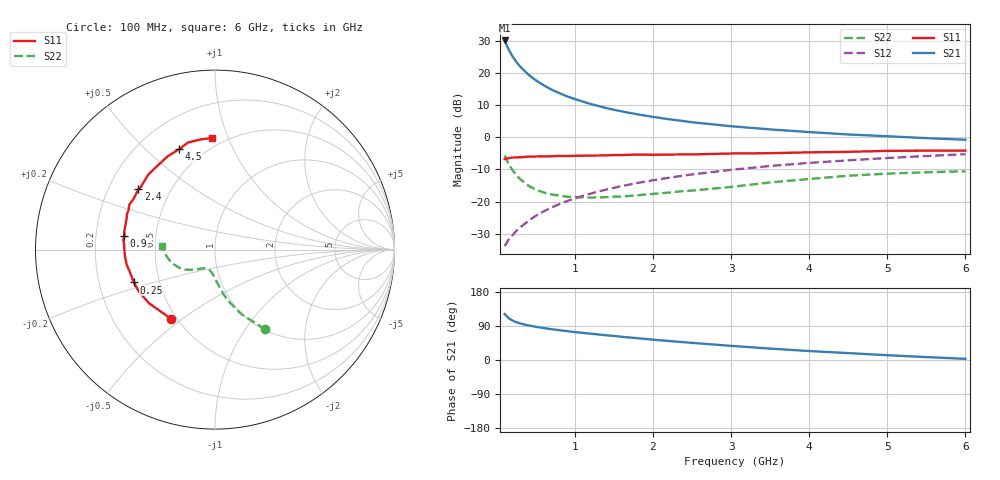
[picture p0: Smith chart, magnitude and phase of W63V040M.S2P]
! SIEMENS Small Signal Semiconductors
! BFR193W
! Si NPN RF Bipolar Junction Transistor in SOT323
! VCE = 3 V  IC = 40 mA
! Common Emitter S-Parameters:  September  1992
# GHz  S  MA  R  50
!  f  S11  S21  S12  S22
! GHz  MAG  ANG  MAG  ANG  MAG  ANG  MAG  ANG
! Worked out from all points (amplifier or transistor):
!   28 points, 100 MHz to 6 GHz, reference 50 ohm
!   highest |S21| = 30.2 dB at 100 MHz (marker M1)
!   |S21| within 3 dB of that: start of sweep to 156.1 MHz
!   unconditionally stable (mu >= 1): 556.4 MHz to 2.38 GHz; 2.431 GHz to 2.542 GHz
!   at 300 MHz: K = 0.90, MSG = 25.0 dB, |S12| = -28.0 dB
!   at 1.5 GHz: K = 1.03, MAG = 11.1 dB, |S12| = -15.7 dB
!   at 6 GHz: K = 0.92, MSG = 2.2 dB, |S12| = -5.3 dB
!   S11 on the Smith chart (normalised r, x): 100 MHz: 0.47, -0.46; 250 MHz: 0.36, -0.17; 900 MHz: 0.32, +0.07; 2.4 GHz: 0.33, +0.31; 4.5 GHz: 0.37, +0.64; 6 GHz: 0.43, +0.88
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0.1  0.4569 -122.2  32.18 121.4  0.0202 60.0  0.5249 -57.8
0.15  0.4739 -141.0  23.49 110.8  0.0254 60.5  0.3886 -67.8
0.2  0.4841 -151.0  18.31 104.2  0.0297 62.5  0.3096 -74.1
0.25  0.4877 -158.0  14.93 99.8  0.0349 64.3  0.2562 -79.0
0.3  0.4887 -163.2  12.61 96.4  0.0396 66.2  0.223 -81.9
0.4  0.4993 -170.6  9.556 91.4  0.0494 68.9  0.1781 -87.1
0.5  0.5026 -175.5  7.703 87.6  0.06 70.4  0.1527 -91.1
0.6  0.5051 -179.7  6.453 84.3  0.0703 71.3  0.1383 -95.4
0.7  0.5069 177.0  5.53 81.3  0.0806 71.7  0.1291 -98.2
0.8  0.5134 173.9  4.87 78.7  0.0909 71.8  0.1239 -101.5
0.9  0.5115 171.2  4.339 76.2  0.1018 71.7  0.1187 -103.9
1  0.5157 168.6  3.935 73.7  0.1122 71.4  0.1175 -106.1
1.2  0.5179 163.8  3.303 69.5  0.1328 70.6  0.1153 -112.0
1.4  0.524 159.7  2.857 65.3  0.1534 69.5  0.117 -116.0
1.6  0.5294 155.6  2.533 61.3  0.174 68.3  0.1195 -120.0
2.2  0.5379 144.8  1.915 50.2  0.2344 63.9  0.1378 -128.5
2.4  0.5425 141.8  1.785 46.8  0.2546 62.3  0.1462 -131.2
3  0.5597 131.5  1.487 37.3  0.3115 57.3  0.169 -138.2
3.5  0.5662 124.8  1.327 30.1  0.3581 52.9  0.1984 -145.7
4.5  0.594 109.5  1.107 18.2  0.438 44.1  0.2524 -162.8
5.5  0.6194 96.9  0.97 7.7  0.5114 35.5  0.2857 -179.1
6  0.6223 91.3  0.916 3.1  0.5461 31.1  0.2963 176.3
